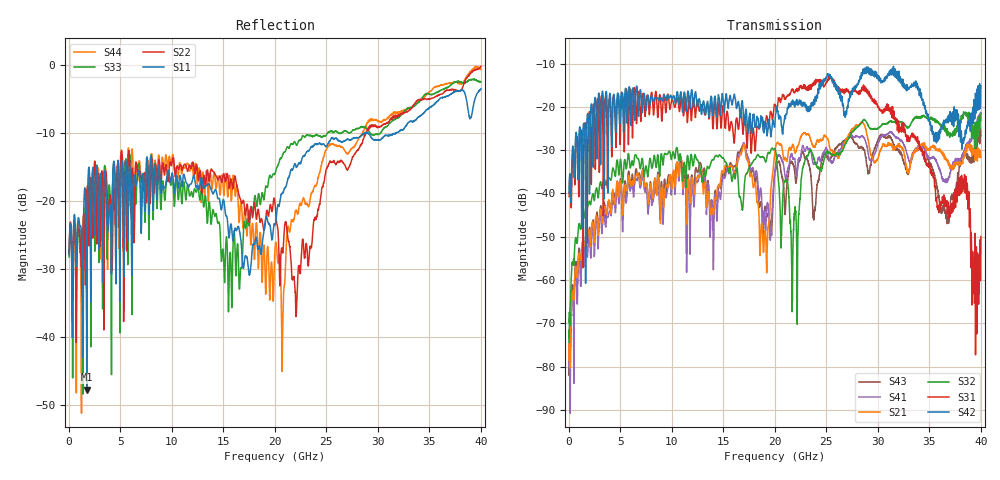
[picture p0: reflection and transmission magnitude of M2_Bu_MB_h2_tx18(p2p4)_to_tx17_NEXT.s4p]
! S11 = S11
! S12 = S12
! S13 = S13
! S14 = S14
! S21 = S21
! S22 = S22
! S23 = S23
! S24 = S24
! S31 = S31
! S32 = S32
! S33 = S33
! S34 = S34
! S41 = S41
! S42 = S42
! S43 = S43
! S44 = S44
! FILE: \\englab.brocade.com\shares\Groups\SIT\Work\Shaohua\IEEE_channels\M2_Bu_MB_h2_tx18(p2p4)_to_tx17_NEXT.s4p
!$DUT_CFG_DESC: Default 4-Port Configuration
!$NUMBER_PORTS: 4
!$DIFF_PORT_MAP: 1|2P|2|2P|0|UC|0|UC|
!$PORT_MAP: PNA 1|1|<<<<<<|TS 2|2|>>>>>>|PNA 2|3|<<<<<<|TS 4|4|>>>>>>|
# MHz S RI R 50.00
! FREQ  S11  S12  S13  S14
!  S21  S22  S23  S24
!  S31  S32  S33  S34
!  S41  S42  S43  S44
!  REAL  IMAG  REAL  IMAG  REAL  IMAG  REAL  IMAG
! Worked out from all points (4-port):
!   3996 points, 50 MHz to 40 GHz, reference 50 ohm
!   strongest paths, dB at 50 MHz, 10.04 GHz, 20.03 GHz, 30.02 GHz, 40 GHz:
!     S42: -39.8, -18.1, -23.4, -13.0, -15.1
!     S31: -40.7, -18.3, -19.6, -20.0, -50.0
!     S32: -74.4, -31.4, -29.6, -24.9, -21.5
!     S21: -74.0, -38.5, -30.1, -31.9, -30.9
!     S41: -71.7, -37.9, -34.3, -28.6, -21.5
!     S43: -74.2, -36.4, -35.0, -27.8, -26.6
!   lowest |S11| = -47.7 dB at 1.76 GHz (marker M1), VSWR 1.01, Z = 49.6 - j0.0787 ohm
!   |S11| at or under -10 dB: start of sweep to 28.69 GHz; 28.71776 GHz to 28.80807 GHz (90.31 MHz wide, 0.314 % of centre); 29.01 GHz to 31.79 GHz (2.782 GHz wide, 9.15 % of centre)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
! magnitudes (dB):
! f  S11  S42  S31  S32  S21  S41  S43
! 50 MHz  -27.9  -39.8  -40.7  -74.4  -74.0  -71.7  -74.2
! 1.76 GHz  -47.7  -24.0  -32.1  -43.4  -52.0  -53.4  -49.8
! 16.96 GHz  -29.8  -21.4  -25.4  -41.7  -28.8  -28.3  -28.6
! 19.07 GHz  -23.1  -23.5  -24.5  -32.5  -48.7  -47.4  -43.1
! 20.79 GHz  -18.8  -26.0  -17.3  -40.3  -30.6  -32.8  -37.1
! 25.37 GHz  -11.2  -13.0  -12.9  -30.8  -29.8  -32.3  -32.0
! 40 GHz  -3.5  -15.1  -50.0  -21.5  -30.9  -21.5  -26.6
